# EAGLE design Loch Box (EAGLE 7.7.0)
DESIGNER: A. Stummer; GROUP: A. Steinberg Labs; RELEASE_DATE: 2017 July; REV: A; TITLE: Loch Box; TITLE2: Analog Laser PID

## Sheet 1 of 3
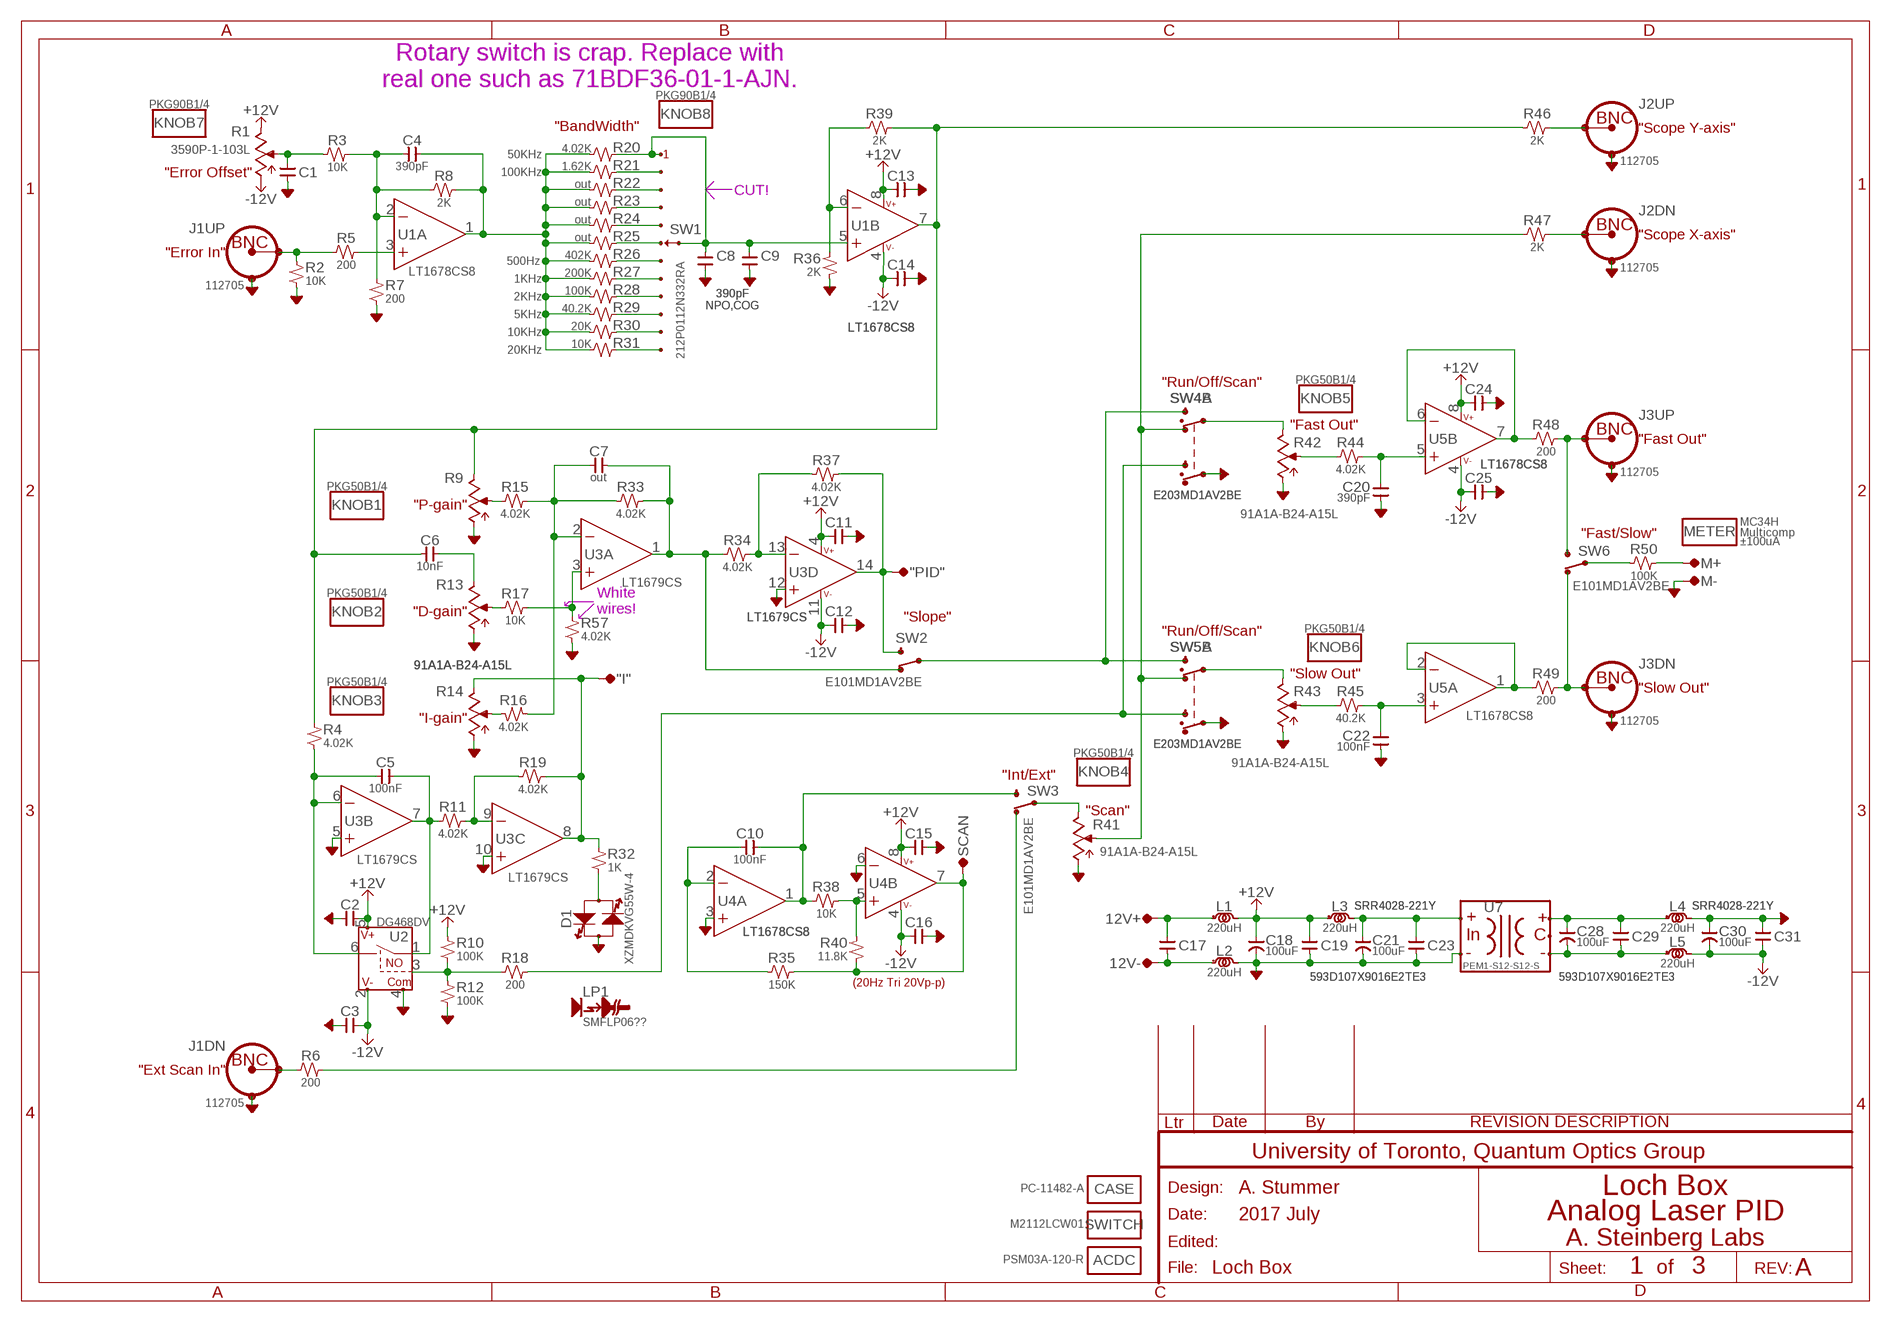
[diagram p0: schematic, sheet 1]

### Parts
12V+  TP-LOOP  [TP-LOOP]
12V-  TP-LOOP  [TP-LOOP]
"I"  TP-0.042B  [TP-0.042B]
"PID"  TP-0.042B  [TP-0.042B]
ACDC  PSM03A-120-R  MISC  [MISC]
C1  100nF  CAP-V-0805  [2012(0805)]
C2  100nF  CAP-H-0805  [2012(0805)]
C3  100nF  CAP-H-0805  [2012(0805)]
C4  390pF  CAP-H-0805  [2012(0805)]
C5  100nF  CAP-H-0805  [2012(0805)]
C6  10nF  CAP-H-0805  [2012(0805)]
C7  out  CAP-H-0805  [2012(0805)]
C8  390pF  CAP-V-0805  [2012(0805)]
C9  390pF  CAP-V-0805  [2012(0805)]
C10  100nF  CAP-H-0805  [2012(0805)]
C11  100nF  CAP-H-0805  [2012(0805)]
C12  100nF  CAP-H-0805  [2012(0805)]
C13  100nF  CAP-H-0805  [2012(0805)]
C14  100nF  CAP-H-0805  [2012(0805)]
C15  100nF  CAP-H-0805  [2012(0805)]
C16  100nF  CAP-H-0805  [2012(0805)]
C17  100nF  CAP-V-0805  [2012(0805)]
C18  100uF  CAP-POL-2917(7343)  [2917(7343)]
C19  100nF  CAP-V-0805  [2012(0805)]
C20  390pF  CAP-V-0805  [2012(0805)]
C21  100uF  CAP-POL-2917(7343)  [2917(7343)]
C22  100nF  CAP-V-0805  [2012(0805)]
C23  100nF  CAP-V-0805  [2012(0805)]
C24  100nF  CAP-H-0805  [2012(0805)]
C25  100nF  CAP-H-0805  [2012(0805)]
C28  100uF  CAP-POL-2917(7343)  [2917(7343)]
C29  100nF  CAP-V-0805  [2012(0805)]
C30  100uF  CAP-POL-2917(7343)  [2917(7343)]
C31  100nF  CAP-V-0805  [2012(0805)]
CASE  PC-11482-A  MISC  [MISC]
D1  XZMDKVG55W-4  LED,DUAL(BIPOLAR)-1206  [1206(3216)]
J1  112705  CONN:BNC,DUAL-112705_ETC  [CONN:BNC,DUAL(BOMAR)]
J2  112705  CONN:BNC,DUAL-112705_ETC  [CONN:BNC,DUAL(BOMAR)]
J3  112705  CONN:BNC,DUAL-112705_ETC  [CONN:BNC,DUAL(BOMAR)]
KNOB1  PKG50B1/4  MISC  [MISC]
KNOB2  PKG50B1/4  MISC  [MISC]
KNOB3  PKG50B1/4  MISC  [MISC]
KNOB4  PKG50B1/4  MISC  [MISC]
KNOB5  PKG50B1/4  MISC  [MISC]
KNOB6  PKG50B1/4  MISC  [MISC]
KNOB7  PKG90B1/4  MISC  [MISC]
KNOB8  PKG90B1/4  MISC  [MISC]
L1  220uH  INDUCTOR-WURTH_744  [INDUCTOR:WURTH_74405]
L2  220uH  INDUCTOR-WURTH_744  [INDUCTOR:WURTH_74405]
L3  220uH  INDUCTOR-WURTH_744  [INDUCTOR:WURTH_74405]
L4  220uH  INDUCTOR-WURTH_744  [INDUCTOR:WURTH_74405]
L5  220uH  INDUCTOR-WURTH_744  [INDUCTOR:WURTH_74405]
LP1  SMFLP06??  LIGHTPIPE-BIVAR_SMFLP  [LIGHTPIPE,BIVAR_SMFLP]
M+  TP-0.042B  [TP-0.042B]
M-  TP-0.042B  [TP-0.042B]
METER  MC34H  MISC  [MISC]
R1  3590P-1-103L  POT-3590  [BOURNS_3590]
R2  10K  R-V-0805  [2012(0805)]
R3  10K  R-H-0805  [2012(0805)]
R4  4.02K  R-V-0805  [2012(0805)]
R5  200  R-H-0805  [2012(0805)]
R6  200  R-H-0805  [2012(0805)]
R7  200  R-V-0805  [2012(0805)]
R8  2K  R-H-0805  [2012(0805)]
R9  91A1A-B24-A15L  POT-BOURNS_91  [BOURNS_91]
R10  100K  R-V-0805  [2012(0805)]
R11  4.02K  R-H-0805  [2012(0805)]
R12  100K  R-V-0805  [2012(0805)]
R13  91A1A-B24-A15L  POT-BOURNS_91  [BOURNS_91]
R14  91A1A-B24-A15L  POT-BOURNS_91  [BOURNS_91]
R15  4.02K  R-H-0805  [2012(0805)]
R16  4.02K  R-H-0805  [2012(0805)]
R17  10K  R-H-0805  [2012(0805)]
R18  200  R-H-0805  [2012(0805)]
R19  4.02K  R-H-0805  [2012(0805)]
R20  4.02K  R-H-0805  [2012(0805)]
R21  1.62K  R-H-0805  [2012(0805)]
R22  out  R-H-0805  [2012(0805)]
R23  out  R-H-0805  [2012(0805)]
R24  out  R-H-0805  [2012(0805)]
R25  out  R-H-0805  [2012(0805)]
R26  402K  R-H-0805  [2012(0805)]
R27  200K  R-H-0805  [2012(0805)]
R28  100K  R-H-0805  [2012(0805)]
R29  40.2K  R-H-0805  [2012(0805)]
R30  20K  R-H-0805  [2012(0805)]
R31  10K  R-H-0805  [2012(0805)]
R32  1K  R-V-0805  [2012(0805)]
R33  4.02K  R-H-0805  [2012(0805)]
R34  4.02K  R-H-0805  [2012(0805)]
R35  150K  R-H-0805  [2012(0805)]
R36  2K  R-V-0805  [2012(0805)]
R37  4.02K  R-H-0805  [2012(0805)]
R38  10K  R-H-0805  [2012(0805)]
R39  2K  R-H-0805  [2012(0805)]
R40  11.8K  R-V-0805  [2012(0805)]
R41  91A1A-B24-A15L  POT-BOURNS_91  [BOURNS_91]
R42  91A1A-B24-A15L  POT-BOURNS_91  [BOURNS_91]
R43  91A1A-B24-A15L  POT-BOURNS_91  [BOURNS_91]
R44  4.02K  R-H-0805  [2012(0805)]
R45  40.2K  R-H-0805  [2012(0805)]
R46  2K  R-H-0805  [2012(0805)]
R47  2K  R-H-0805  [2012(0805)]
R48  200  R-H-0805  [2012(0805)]
R49  200  R-H-0805  [2012(0805)]
R50  100K  R-H-0805  [2012(0805)]
R57  4.02K  R-V-0805  [2012(0805)]
SCAN  TP-0.042B  [TP-0.042B]
SW1  212P0112N332RA  SWITCH,SP12T-CTS_212P0112  [SWITCH,CTS_SP12T(212P0112)]
SW2  E101MD1AV2BE  SWITCH:SPDT-ESWITCH_1??AV2?  [SWITCH:E-SWITCH_1??AV2?]
SW3  E101MD1AV2BE  SWITCH:SPDT-ESWITCH_1??AV2?  [SWITCH:E-SWITCH_1??AV2?]
SW4  E203MD1AV2BE  SWITCH:DPDT-ESWITCH_2??D?AV2?  [SWITCH:E-SWITCH_2??D?AV2?]
SW5  E203MD1AV2BE  SWITCH:DPDT-ESWITCH_2??D?AV2?  [SWITCH:E-SWITCH_2??D?AV2?]
SW6  E101MD1AV2BE  SWITCH:SPDT-ESWITCH_1??AV2?  [SWITCH:E-SWITCH_1??AV2?]
SWITCH  M2112LCW01  MISC  [MISC]
U1  LT1678CS8  OPAMP:AD8___(DUAL)-SOIC-8  [SOIC-8]
U2  DG468DV  SWITCH,ANALOG,SPST,BIPOLAR-TSOP6  [TSOP-6]
U3  LT1679CS  OPAMP,QUAD-SO14  [SOIC-14]
U4  LT1678CS8  OPAMP:AD8___(DUAL)-SOIC-8  [SOIC-8]
U5  LT1678CS8  OPAMP:AD8___(DUAL)-SOIC-8  [SOIC-8]
U7  PEM1-S12-S12-S  DC-DC:DCH01(ISO,UNI/BI,1W)  [DC-DC:DCH01(ISO,UNI/BI,1W)]

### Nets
+12V [power]: C2.1 C11.1 C13.1 C15.1 C18.+(POS) C19.2 C24.1 L1.2(B) L3.1(A) R1.CW R10.2 U1.8(PWR:V++) U2.5(V+) U3.4(V++) U4.8(PWR:V++) U5.8(PWR:V++)
-12V [power]: C3.1 C12.1 C14.1 C16.1 C25.1 C30.-(NEG) C31.1 L5.2(B) R1.CCW U1.4(PWR:V-) U2.2(V-) U3.11(V-) U4.4(PWR:V-) U5.4(PWR:V-)
AGND: C1.1 C2.2 C3.2 C8.1 C9.1 C11.2 C12.2 C13.2 C14.2 C15.2 C16.2 C18.-(NEG) C19.1 C20.1 C21.-(NEG) C22.1 C23.1 C24.2 C25.2 C30.+(POS) C31.2 D1.ONE J1.LWR-COM(DN:SHIELD2) J1.UPR-COM(UP:SHIELD2) J2.LWR-COM(DN:SHIELD2) J2.UPR-COM(UP:SHIELD2) J3.LWR-COM(DN:SHIELD2) J3.UPR-COM(UP:SHIELD2) L2.2(B) L4.2(B) M-.TP R2.1 R7.1 R9.CCW R12.1 R13.CCW R14.CCW R36.1 R41.CCW R42.CCW R43.CCW R57.1 SW4.COM2(B:COM) SW5.COM2(B:COM) U2.4(COM) U3.5(B:+IN) U3.10(C:+IN) U3.12(D:+IN) U4.3(A:+IN) U4.6(B:-IN) U7.IN-
N$1: J1.UPR-CTR(UP:CONDUCTOR) R2.2 R5.1
N$2: R5.2 U1.3(A:+IN)
N$3: C4.1 R3.2 R7.2 R8.1 U1.2(A:-IN)
N$4: C1.2 R1.W R3.1
N$5: C4.2 R8.2 R20.1 R21.1 R22.1 R23.1 R24.1 R25.1 R26.1 R27.1 R28.1 R29.1 R30.1 R31.1 U1.1(A:OUT)
N$6: C6.1 R4.2 R9.CW R39.2 R46.1 U1.7(B:OUT)
N$7: R31.2 SW1.12
N$8: R30.2 SW1.11
N$9: R29.2 SW1.10
N$10: R28.2 SW1.9
N$11: R27.2 SW1.8
N$12: R26.2 SW1.7
N$13: R25.2 SW1.6
N$14: R24.2 SW1.5
N$15: R23.2 SW1.4
N$16: R22.2 SW1.3
N$17: R21.2 SW1.2
N$18: C8.2 C9.2 R20.2 SW1.1 SW1.D(W) U1.5(B:+IN)
N$19: J2.UPR-CTR(UP:CONDUCTOR) R46.2
N$20: R36.2 R39.1 U1.6(B:-IN)
N$21: R9.WIPER(W) R15.1
N$22: R13.WIPER(W) R17.1
N$23: C6.2 R13.CW
N$24: SW2.COM SW4.UP1(A:NO\UP\RIGHT) SW5.UP1(A:NO\UP\RIGHT)
N$25: C7.2 R33.2 R34.1 SW2.DOWN(NC\DOWN\LEFT) U3.1(A:OUT)
N$26: R34.2 R37.1 U3.13(D:-IN)
N$27: C7.1 R15.2 R16.1 R33.1 U3.2(A:-IN)
N$28: "PID".TP R37.2 SW2.UP(NO\UP\RIGHT) U3.14(D:OUT)
N$29: C5.1 R4.1 U2.6(SW2) U3.6(B:-IN)
N$30: C5.2 R11.1 U2.1(SW1) U3.7(B:OUT)
N$31: R11.2 R19.1 U3.9(C:-IN)
N$32: "I".TP R14.CW R19.2 R32.2 U3.8(C:OUT)
N$33: R18.2 SW4.UP2(B:NO\UP\RIGHT) SW5.UP2(B:NO\UP\RIGHT)
N$34: R14.WIPER(W) R16.2
N$35: R41.WIPER(W) R47.1 SW4.DN1(A:NC\DOWN\LEFT) SW5.DN1(A:NC\DOWN\LEFT)
N$36: R42.CW SW4.COM1(A:COM)
N$37: R48.1 U5.6(B:-IN) U5.7(B:OUT)
N$38: R42.WIPER(W) R44.1
N$39: C20.2 R44.2 U5.5(B:+IN)
N$40: J3.UPR-CTR(UP:CONDUCTOR) R48.2 SW6.UP(NO\UP\RIGHT)
N$41: R10.1 R12.2 R18.1 U2.3(IN)
N$42: R38.2 R40.2 U4.5(B:+IN)
N$43: R43.CW SW5.COM1(A:COM)
N$44: R49.1 U5.1(A:OUT) U5.2(A:-IN)
N$45: R43.WIPER(W) R45.1
N$46: C22.2 R45.2 U5.3(A:+IN)
N$47: J3.LWR-CTR(DN:CONDUCTOR) R49.2 SW6.DOWN(NC\DOWN\LEFT)
N$48: C10.1 R35.1 U4.2(A:-IN)
N$49: R41.CW SW3.COM
N$50: J1.LWR-CTR(DN:CONDUCTOR) R6.1
N$51: C10.2 R38.1 SW3.UP(NO\UP\RIGHT) U4.1(A:OUT)
N$52: R50.1 SW6.COM
N$53: R6.2 SW3.DOWN(NC\DOWN\LEFT)
N$54: J2.LWR-CTR(DN:CONDUCTOR) R47.2
N$55: R35.2 R40.1 SCAN.TP U4.7(B:OUT)
N$56: M+.TP R50.2
N$57: D1.T'OTHER R32.1
N$58 [power]: 12V-.P$1(TP) C17.1 L2.1(A)
N$59 [power]: C28.+(POS) C29.2 L4.1(A) U7.OUT+
N$60 [power]: C21.+(POS) C23.2 L3.2(B) U7.IN+
N$62 [power]: 12V+.P$1(TP) C17.2 L1.1(A)
N$64 [power]: C28.-(NEG) C29.1 L5.1(A) U7.OUT-
N$69: R17.2 R57.2 U3.3(A:+IN)
Unconnected: SW4.DN2(B:NC\DOWN\LEFT) SW5.DN2(B:NC\DOWN\LEFT) U7.COM

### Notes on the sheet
- Rotary switch is crap. Replace with
  real one such as 71BDF36-01-1-AJN.
- "Scope Y-axis"
- 50KHz
- "Error Offset" | 100KHz
- CUT!
- "Scope X-axis"
- "Error In"
- 500Hz
- 1KHz
- 2KHz
- 5KHz
- 10KHz
- 20KHz
- "Fast Out"
- White
  wires!
- "Slow Out"
- NO
- (20Hz Tri 20Vp-p)
- "Ext Scan In"

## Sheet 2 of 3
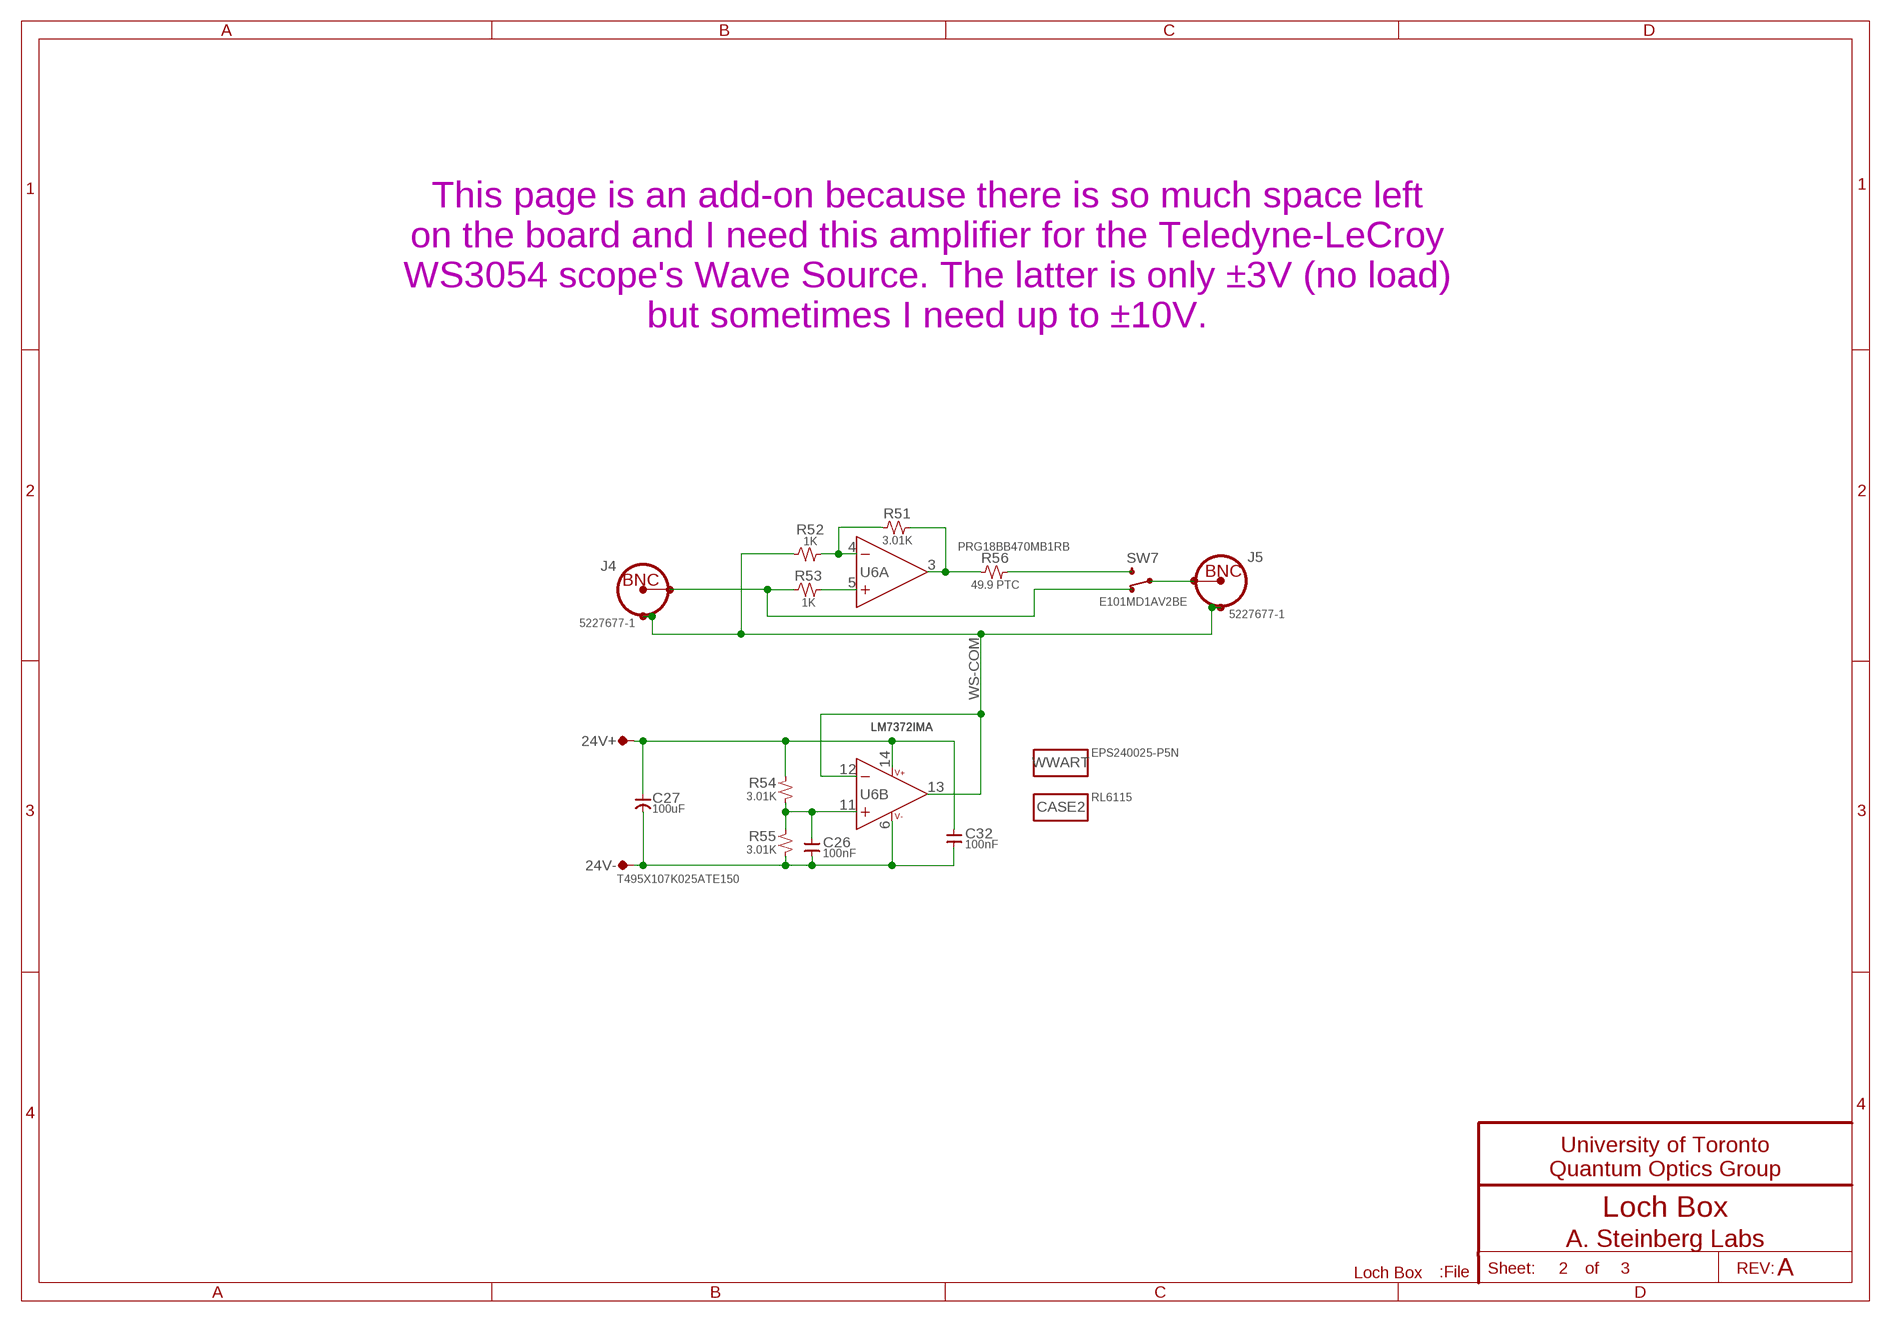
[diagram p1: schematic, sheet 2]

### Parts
24V+  TP-LOOP  [TP-LOOP]
24V-  TP-LOOP  [TP-LOOP]
C26  100nF  CAP-V-0805  [2012(0805)]
C27  100uF  CAP-POL-2917(7343)  [2917(7343)]
C32  100nF  CAP-V-0805  [2012(0805)]
CASE2  RL6115  MISC  [MISC]
J4  5227677-1  CONN:BNCTYPE3HORIZ  [CONN:BNC-AMP-TYPE3HORIZ]
J5  5227677-1  CONN:BNCTYPE3HORIZ  [CONN:BNC-AMP-TYPE3HORIZ]
R51  3.01K  R-H-0805  [2012(0805)]
R52  1K  R-H-0805  [2012(0805)]
R53  1K  R-H-0805  [2012(0805)]
R54  3.01K  R-V-0805  [2012(0805)]
R55  3.01K  R-V-0805  [2012(0805)]
R56  49.9 PTC  R-H-0805  [2012(0805)]
SW7  E101MD1AV2BE  SWITCH:SPDT-ESWITCH_1??AV2?  [SWITCH:E-SWITCH_1??AV2?]
U6  LM7372IMA  OPAMP_DUAL-SOIC16#1  [SOIC-16]
WWART  EPS240025-P5N  MISC  [MISC]

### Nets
N$63: R51.1 R52.2 U6.4(A:-IN)
N$65: R56.2 SW7.UP(NO\UP\RIGHT)
N$66: J5.CONDUCTOR SW7.COM
N$67: J4.CONDUCTOR R53.1 SW7.DOWN(NC\DOWN\LEFT)
N$68: R53.2 U6.5(A:+IN)
N$70: C26.2 R54.1 R55.2 U6.11(B:+IN)
N$71: 24V-.P$1(TP) C26.1 C27.-(NEG) C32.1 R55.1 U6.6(.:V-)
N$72: 24V+.P$1(TP) C27.+(POS) C32.2 R54.2 U6.14(.:V++)
N$74: R51.2 R56.1 U6.3(A:OUT)
WS-COM: J4.SHIELD1 J4.SHIELD2 J5.SHIELD1 J5.SHIELD2 R52.1 U6.12(B:-IN) U6.13(B:OUT)

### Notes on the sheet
- This page is an add-on because there is so much space left
  on the board and I need this amplifier for the Teledyne-LeCroy
  WS3054 scope's Wave Source. The latter is only ±3V (no load)
  but sometimes I need up to ±10V.

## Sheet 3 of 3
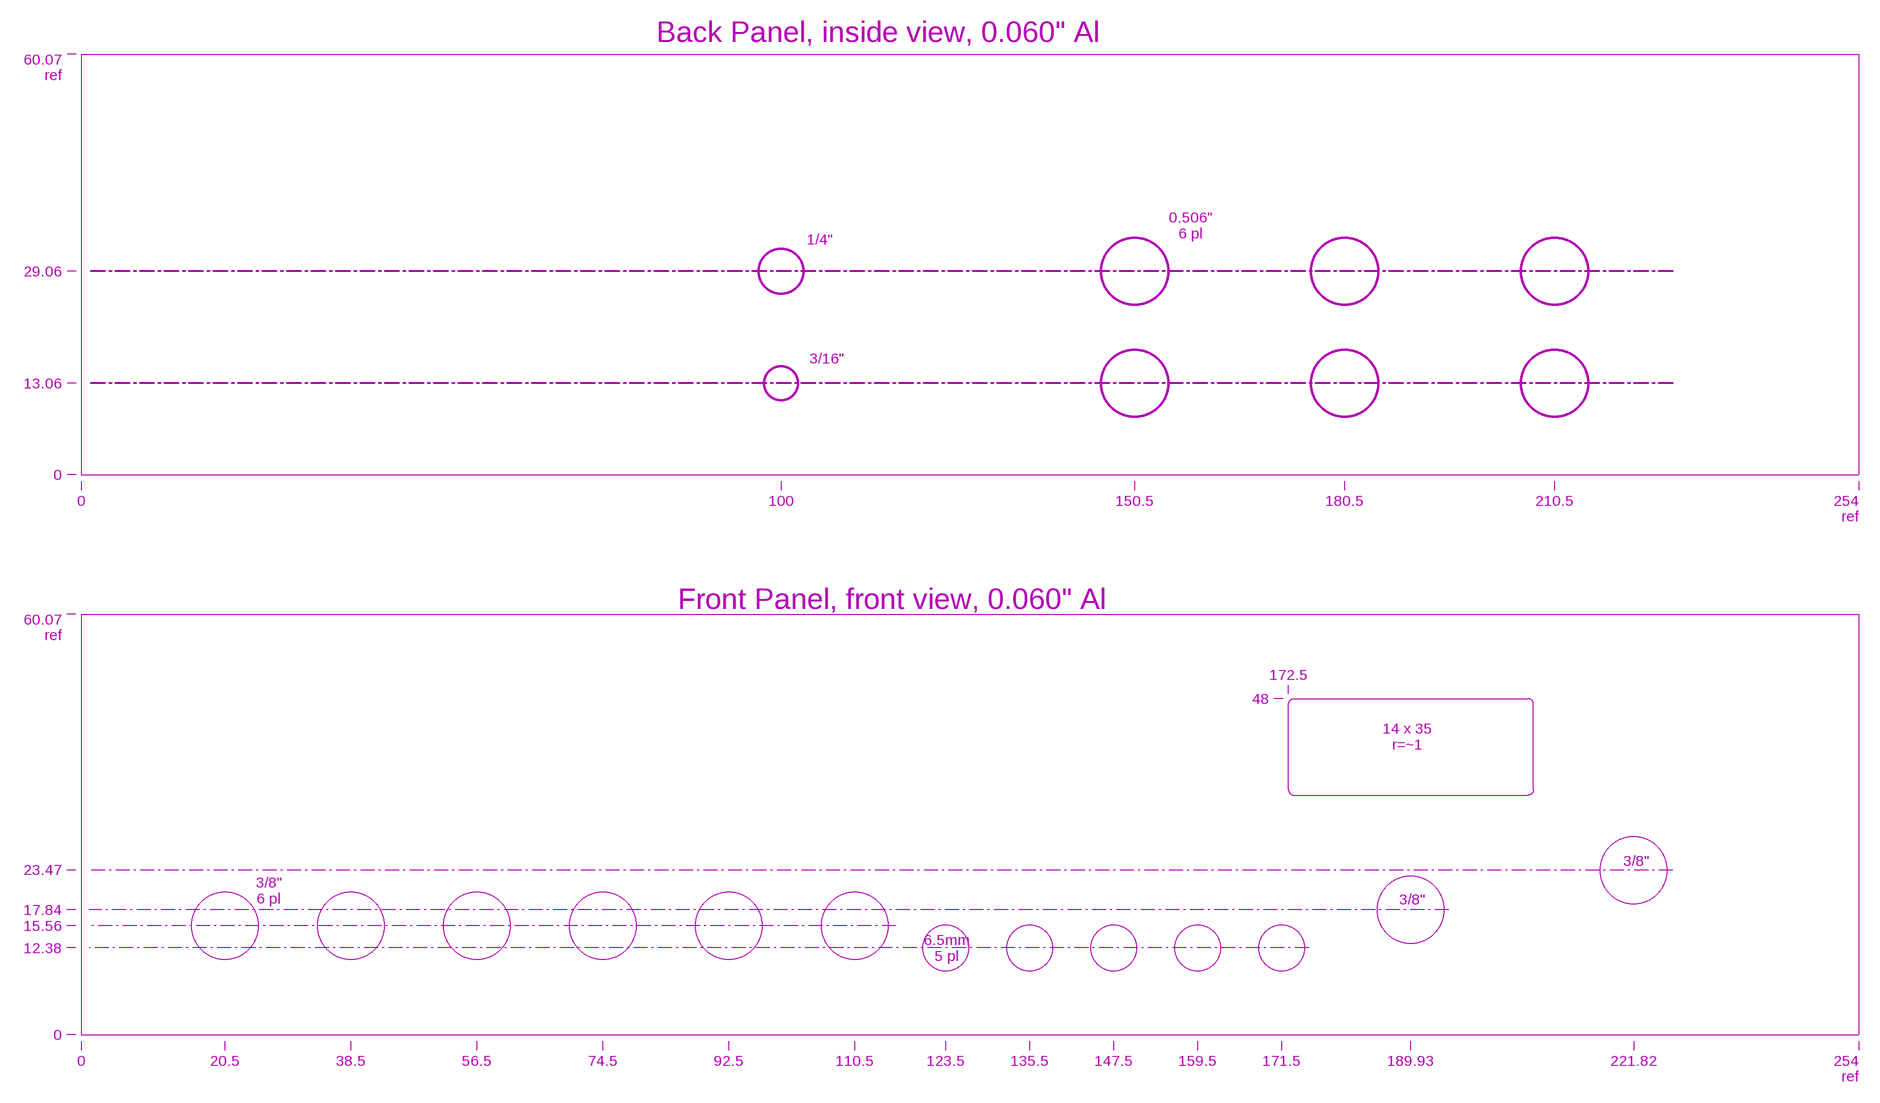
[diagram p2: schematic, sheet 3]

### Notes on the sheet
- Back Panel, inside view, 0.060" Al
- 60.07
  ref
- 0.506"
  6 pl
- 1/4"
- 29.06
- 3/16"
- 13.06
- 0
- 0 | 100 | 150.5 | 180.5 | 210.5
- 254
  ref
- Front Panel, front view, 0.060" Al
- 60.07
  ref
- 172.5
- 48
- 14 x 35
  r=~1
- 3/8"
- 23.47
- 3/8"
  6 pl
- 3/8"
- 17.84
- 15.56
- 6.5mm
  5 pl
- 12.38
- 0
- 0 | 20.5 | 38.5 | 56.5 | 74.5 | 92.5 | 110.5 | 123.5 | 135.5 | 147.5 | 159.5 | 171.5 | 189.93 | 221.82
- 254
  ref

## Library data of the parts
12V+ 12V- 24V+ 24V- "I" "PID" M+ M- SCAN = QuantumOptics:TP: Testpoint, single pin or single socket, either SMT pad, small hole or loop style TP such as Keystone 5002K (0.042").
ACDC CASE CASE2 KNOB1-KNOB8 SWITCH WWART = QuantumOptics:MISC: Miscellaneous Part, just a placeholder for miscellaeous parts
C1 C17 C19 C20 C22 C23 C26 C29 C31 C32 = QuantumOptics:CAP-V-: Cap, SMT and Through-hole, 0402 and up.
C2-C7 C10-C16 C24 C25 = QuantumOptics:CAP-H-: Cap, SMT and Through-hole, 0402 and up.
C8 C9 = QuantumOptics:CAP-V-: Cap, SMT and Through-hole, 0402 and up.; TEMPCO: NPO,COG
C18 C21 C28 C30 = QuantumOptics:CAP-POL-: Capacitor, Polarized, SMT 0805 and up, probably tantalum.; PN: 593D107X9016E2TE3
C27 = QuantumOptics:CAP-POL-: Capacitor, Polarized, SMT 0805 and up, probably tantalum.; PN: T495X107K025ATE150
D1 = QuantumOptics:LED,DUAL(BIPOLAR): LED, dual biploar such as SunLED XZMDKVG55W-4.
J1-J3 = QuantumOptics:CONN:BNC,DUAL: Dual BNC, panel mount RA throughhole, Isolated: Amphenol 31-657 and 112705/6. Sheilds connected: Amphenol 031-6578, Cinch VBI501 (cheapest) and Bomar 364A2595.; NUT: 1-1634816-0
J4 J5 = QuantumOptics:CONN:BNC: BNC PCB, horizontal or vertical, e.g. Horiz: Amp (5)227677-1, nut 1-329631-2, shoulder washer 330620, vert isolated 5227222-6, http://catalog.tycoelectronics.com/TE/bin/TE.Connect?C=1&M=BYPN&TCPN=5227222-6&RQPN=5227222-6 ...
L1-L5 = QuantumOptics:INDUCTOR: Inductor, generic inductor.; PN: SRR4028-221Y
LP1 = QuantumOptics:LIGHTPIPE: Lightpipe for SMT LEDs
METER = QuantumOptics:MISC: Miscellaneous Part, just a placeholder for miscellaeous parts; MFG: Multicomp; RANGE: ±100uA
R1 = QuantumOptics:POT: Pot, regular or trimpot
R2 R4 R7 R10 R12 R32 R36 R40 R54 R55 R57 = QuantumOptics:R-V-*: Resistor, SMT & Through-Hole, vertical symbol
R3 R5 R6 R8 R11 R15-R31 R33-R35 R37-R39 R44-R53 = QuantumOptics:R-H-*: Resistor, SMT & Through-Hole, horizontal symbol
R9 = QuantumOptics:POT: Pot, regular or trimpot; DESC: "P-gain"
R13 = QuantumOptics:POT: Pot, regular or trimpot; DESC: "D-gain"
R14 = QuantumOptics:POT: Pot, regular or trimpot; DESC: "I-gain"
R41 = QuantumOptics:POT: Pot, regular or trimpot; DESC: "Scan"
R42 = QuantumOptics:POT: Pot, regular or trimpot; DESC: "Fast Out"
R43 = QuantumOptics:POT: Pot, regular or trimpot; DESC: "Slow Out"
R56 = QuantumOptics:R-H-*: Resistor, SMT & Through-Hole, horizontal symbol; PN: PRG18BB470MB1RB
SW1 = QuantumOptics:SWITCH,SP12T: Switch, SP12T, can be part of DP12T, can have stops to reduce positions.; DESC: "BandWidth"
SW2 = QuantumOptics:SWITCH:SPDT: Switch, SPDT; DESC: "Slope"
SW3 = QuantumOptics:SWITCH:SPDT: Switch, SPDT; DESC: "Int/Ext"
SW4 SW5 = QuantumOptics:SWITCH:DPDT: Switch, DPDT; DESC: "Run/Off/Scan"
SW6 = QuantumOptics:SWITCH:SPDT: Switch, SPDT; DESC: "Fast/Slow"
SW7 = QuantumOptics:SWITCH:SPDT: Switch, SPDT
U1 U4 U5 = QuantumOptics:OPAMP:AD8___(DUAL): AD8xxx, Analog Devices, dual opamp in SOIC-8 and MSOP-8, various versions available. AD8066, AD8656, etc. e.g. http://www.analog.com/UploadedFiles/Data_Sheets/476080131AD8655_6_a.pdf
U2 = QuantumOptics:SWITCH,ANALOG,SPST,BIPOLAR: Analog SPST switch, bipolar such as Vishay DG467/8
U3 = QuantumOptics:OPAMP,QUAD: Quad opamp, such as LT1679 or LT1491
U6 = QuantumOptics:OPAMP_DUAL: Dual Op Amp, common pinouts. Based on http://www.analog.com/static/imported-files/data_sheets/AD8651_8652.pdf
U7 = QuantumOptics:DC-DC:DCH01(ISO,UNI/BI,1W): DC-DC DCH01, TI, isolated, unregulated, uni- bipolar. http://focus.ti.com/lit/ds/symlink/dch010505d.pdf; MFG: TI

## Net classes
0 default: width 0.152 mm, drill 0.254 mm, clearance 0.152 mm
1 power: width 0.635 mm, drill 0.254 mm, clearance 0.254 mm

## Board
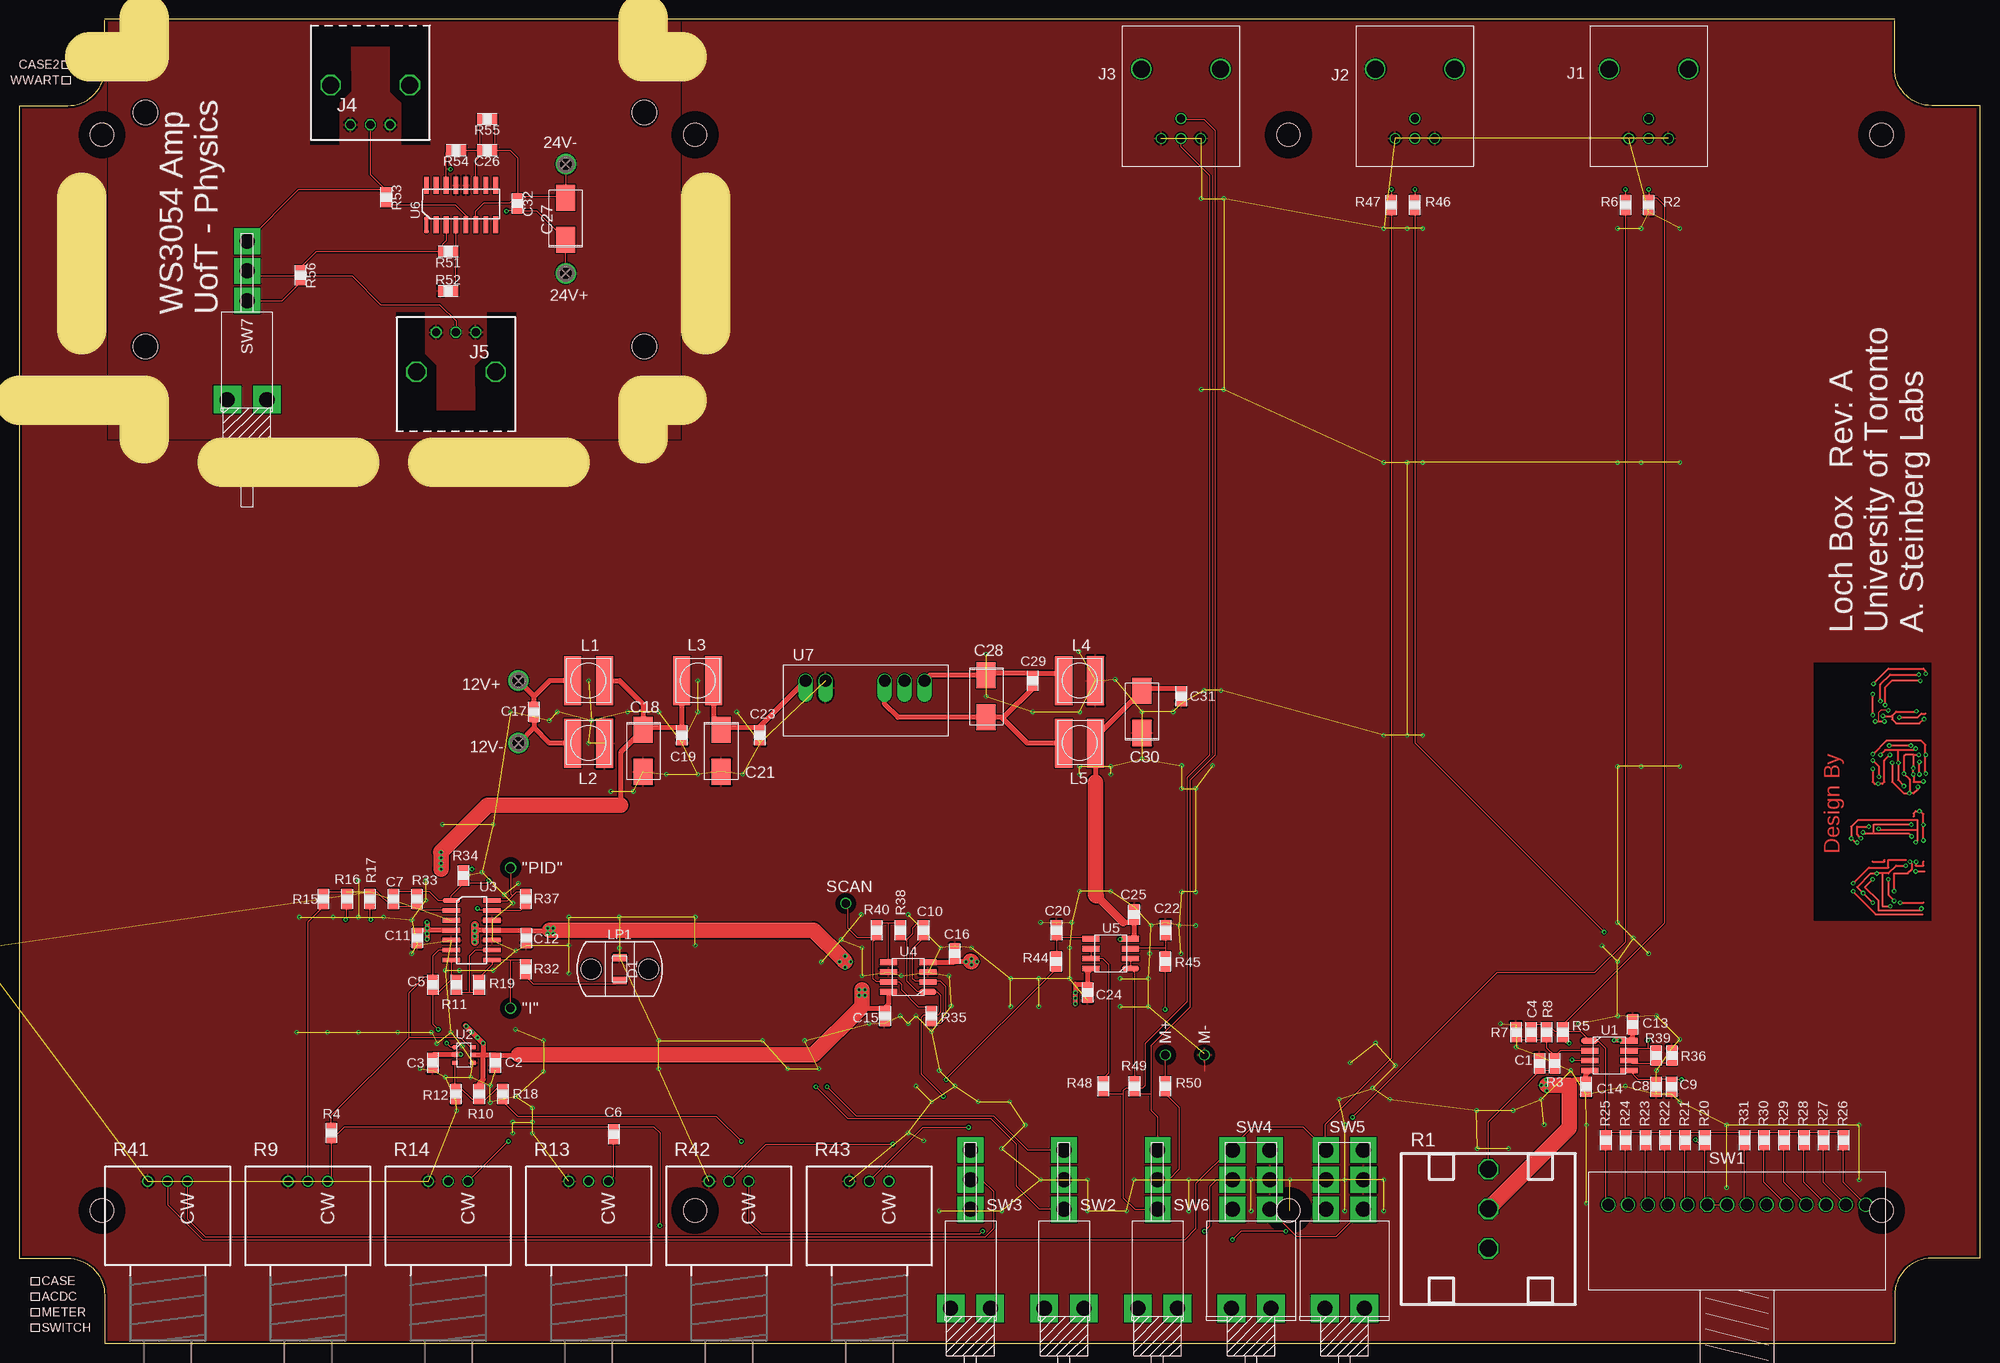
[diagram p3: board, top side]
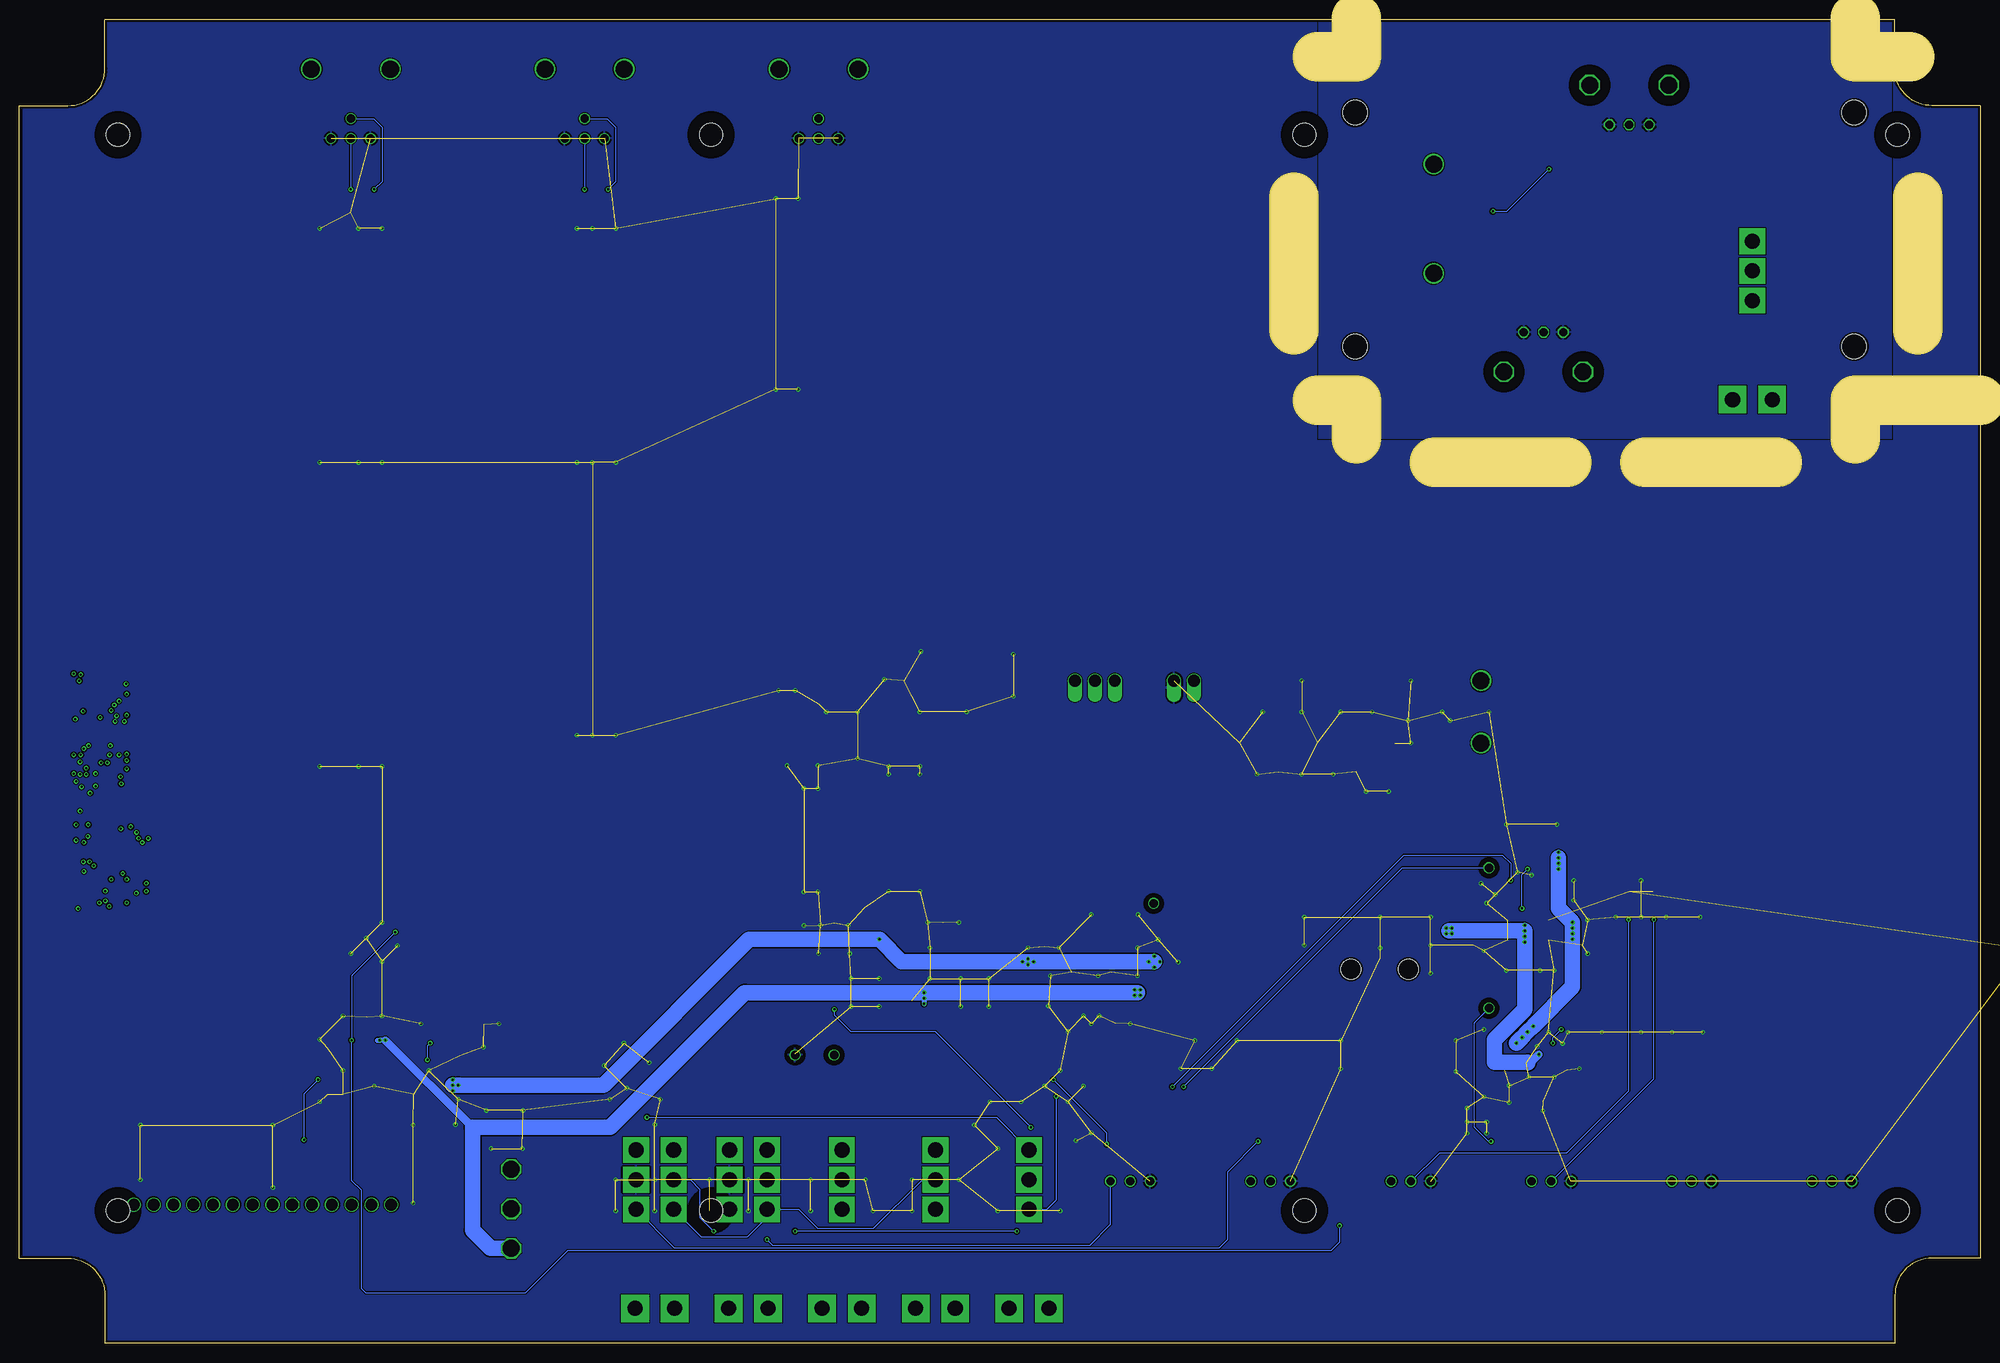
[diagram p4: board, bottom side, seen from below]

Size 251.5 x 169.8 mm. Coordinates in mm from the lower left corner, seen from the top.
Copper layers (1+16): Top 0.04318125mm / dielectric 7.5mil / Bottom 0.04318125mm
Design rules "~DRC for PCBWay, 2-layer #1, 6&6mil & 0.3mm drill": minimum track width 6mil, minimum drill 0.25mm, track to track 6mil, track to pad 6mil, pad to pad 6mil, via to via 6mil, smd to smd 0mil, copper to edge 10mil, drill to drill 6mil, minimum pad ring 6mil, minimum via ring 6mil, stop-mask expansion 4mil, vias tented up to drill 0mil, thermal gap 10mil
Holes 3.17 mm at 16.14,127.85 16.14,157.85 80.15,157.85 80.15,127.85
tRestrict: 4 lines
Milling: 12 lines

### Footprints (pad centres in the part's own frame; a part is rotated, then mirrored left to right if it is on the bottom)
TP-LOOP = drill 2.184 pad 2.54: P$1 0,0
TP-0.042B = drill 1.092: TP 0,0
2012(0805) = smd 0.7 x 1.3: 1 -0.95,0; 2 0.95,0
2917(7343) = smd 3.35 x 2.45: + -2.7,0; - 2.7,0
1206(3216) = smd 0.9 x 1.7: ONE -1.45,0; T'OTHER 1.45,0
CONN:BNC,DUAL(BOMAR) = drill 1.067: LWR-COM 14.45,-2.54; LWR-CTR 11.91,0; UPR-COM 14.45,2.54; UPR-CTR 14.45,0 | drill 2.184: MTG1 5.56,-5.08; MTG2 5.56,5.08
CONN:BNC-AMP-TYPE3HORIZ = drill 1.067 octagon: CONDUCTOR 0,-12.7; SHIELD1 -2.54,-12.7; SHIELD2 2.54,-12.7 | drill 2.184 octagon: P$1 -5.08,-7.62; P$2 5.08,-7.62
INDUCTOR:WURTH_74405 = smd 6.3 x 2.2: 1 0,2.05; 2 0,-2.05
LIGHTPIPE,BIVAR_SMFLP = hole 2.578: -3.683,0; 3.683,0
BOURNS_3590 = drill 2.184 octagon: CCW -12.065,0; CW -6.985,0; W -17.145,0
BOURNS_91 = drill 1.067: CCW -10.795,-2.54; CW -10.795,2.54; WIPER -10.795,0
SWITCH,CTS_SP12T(212P0112) = drill 1.5: 1 0,-1.27; 2 0,-6.35; 3 0,-8.89; 4 0,-11.43; 5 0,-13.97; 6 0,-16.51; 7 0,16.51; 8 0,13.97; 9 0,11.43; 10 0,8.89; 11 0,6.35; 11.5 0,3.81; 12 0,1.27 | drill 1.5 octagon: D 0,-3.81
SWITCH:E-SWITCH_1??AV2? = drill 1.93 pad 3.302 square: COM 0,0; DOWN -3.81,0; UP 3.81,0 | drill 1.93 pad 3.556 square: MTG1 16.51,-2.54; MTG2 16.51,2.54
SWITCH:E-SWITCH_2??D?AV2? = drill 1.93 pad 3.302 square: COM1 0,-2.413; COM2 0,2.413; DN1 -3.81,-2.413; DN2 -3.81,2.413; UP1 3.81,-2.413; UP2 3.81,2.413 | drill 1.93 pad 3.556 square: MTG1 16.51,-2.54; MTG2 16.51,2.54
SOIC-8 = smd 0.75 x 2.2: 1 -1.905,-2.532; 2 -0.635,-2.532; 3 0.635,-2.532; 4 1.905,-2.532; 5 1.905,2.532; 6 0.635,2.532; 7 -0.635,2.532; 8 -1.905,2.532
TSOP-6 = smd 0.508 x 0.711: 1 -0.991,-1.168; 2 0,-1.168; 3 0.991,-1.168; 4 0.991,1.168; 5 0,1.168; 6 -0.991,1.168
SOIC-14 = smd 0.6 x 2.2: 1 -3.81,-2.6; 2 -2.54,-2.6; 3 -1.27,-2.6; 4 0,-2.6; 5 1.27,-2.6; 6 2.54,-2.6; 7 3.81,-2.6; 8 3.81,2.6; 9 2.54,2.6; 10 1.27,2.6; 11 0,2.6; 12 -1.27,2.6; 13 -2.54,2.6; 14 -3.81,2.6
SOIC-16 = smd 0.6 x 2.2: 1 -3.81,-2.54; 2 -2.54,-2.54; 3 -1.27,-2.54; 4 0,-2.54; 5 1.27,-2.54; 6 2.54,-2.54; 7 3.81,-2.54; 8 5.08,-2.54; 9 5.08,2.54; 10 3.81,2.54; 11 2.54,2.54; 12 1.27,2.54; 13 0,2.54; 14 -1.27,2.54; 15 -2.54,2.54; 16 -3.81,2.54
DC-DC:DCH01(ISO,UNI/BI,1W) = drill 1.524 offset: COM 2.54,0; IN+ -10.16,0; IN- -7.62,0; OUT+ 5.08,0; OUT- 0,0
CASE,BUD_PC11482 = hole 3: 10.582,17.056; 86.681,17.056; 162.779,17.056; 238.878,17.056; 10.582,155.029; 86.681,155.029; 162.779,155.029; 238.878,155.029

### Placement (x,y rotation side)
12V+  64,85 0 top
12V-  64,77 0 top
24V+  70.08,137.24 180 top
24V-  70.08,151.24 0 top
"I"  63,43 0 top
"PID"  63,61 0 top
ACDC  2,6 0 top
C1  194.96,35.92 270 top
C2  61,36 270 top
C3  53,36 270 top
C4  193.96,39.92 90 top
C5  53,46 270 top
C6  76.21,26.84 270 top
C7  48,57 90 top
C8  209.96,32.92 90 top
C9  211.96,32.92 90 top
C10  116,53 90 top
C11  51,52 270 top
C12  65,52 270 top
C13  206.96,40.92 90 top
C14  200.96,32.92 270 top
C15  111,42 270 top
C16  120,50 90 top
C17  66,81 90 top
C18  80,76 270 top
C19  85,78 90 top
C20  133,53 270 top
C21  90,76 270 top
C22  147,53 270 top
C23  95,78 90 top
C24  137,45 270 top
C25  143,55 90 top
C26  60,153 180 top
C27  70.08,144.24 90 top
C28  124,83 270 top
C29  130,85 90 top
C30  144,81 90 top
C31  149,83 270 top
C32  63.84,146.2 270 top
CASE  2,8 0 top
CASE2  6,164 180 top
D1  77,48 270 top
J1  209,169 270 top
J2  179,169 270 top
J3  149,169 270 top
J4  45,169 0 top
J5  56,117 180 top
KNOB1  not placed on the board
KNOB2  not placed on the board
KNOB3  not placed on the board
KNOB4  not placed on the board
KNOB5  not placed on the board
KNOB6  not placed on the board
KNOB7  not placed on the board
KNOB8  not placed on the board
L1  73,85 90 top
L2  73,77 90 top
L3  87,85 90 top
L4  136,85 90 top
L5  136,77 90 top
LP1  77,48 0 top
M+  147,37 90 top
M-  152,37 90 top
METER  2,4 0 top
R1  188.43,5.2 270 top
R2  209,146 90 top
R3  196.96,35.92 90 top
R4  40,27 270 top
R5  197.96,39.92 270 top
R6  206,146 270 top
R7  191.96,39.92 270 top
R8  195.96,39.92 90 top
R9  37,10 270 top
R10  59,32 90 top
R11  56,46 270 top
R12  56,32 90 top
R13  73,10 270 top
R14  55,10 270 top
R15  39,57 90 top
R16  42,57 270 top
R17  45,57 90 top
R18  62,32 270 top
R19  59,46 90 top
R20  216.17,26.05 270 top
R21  213.63,26.05 270 top
R22  211.09,26.05 270 top
R23  208.55,26.05 270 top
R24  206.01,26.05 270 top
R25  203.47,26.05 270 top
R26  233.95,26.05 270 top
R27  231.41,26.05 270 top
R28  228.87,26.05 270 top
R29  226.33,26.05 270 top
R30  223.79,26.05 270 top
R31  221.25,26.05 270 top
R32  65,48 90 top
R33  51,57 90 top
R34  57,60 90 top
R35  117,42 90 top
R36  211.96,36.92 270 top
R37  65,57 90 top
R38  113,53 90 top
R39  209.96,36.92 90 top
R40  110,53 90 top
R41  19,10 270 top
R42  91,10 270 top
R43  109,10 270 top
R44  133,49 90 top
R45  147,49 90 top
R46  179,146 90 top
R47  176,146 90 top
R48  139,33 270 top
R49  143,33 270 top
R50  147,33 90 top
R51  55,140 180 top
R52  55,135 0 top
R53  47,147 270 top
R54  56,153 180 top
R55  60,157 180 top
R56  36,137 270 top
R57  not placed on the board
SCAN  106,56.44 0 top
SW1  220.32,17.8 270 top
SW2  134,21 270 top
SW3  122,21 270 top
SW4  158,21 270 top
SW5  170,21 270 top
SW6  146,21 270 top
SW7  29.2,137.56 270 top
SWITCH  2,2 0 top
U1  203.96,36.92 270 top
U2  57,37 270 top
U3  58,53 270 top
U4  114,47 90 top
U5  140,50 90 top
U6  56,146 0 top
U7  111,85 0 top
U$34  [CASE,HAMMOND_RL6105_RL6115]  85,116 90 top
U$47  [CASE,BUD_PC11482]  0,0 0 top
WWART  6,162 180 top

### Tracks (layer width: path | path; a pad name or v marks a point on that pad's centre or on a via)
+12V  (via drill 0.25)
  Top 0.635: C13.1 206.96,39.29 U1.8 206.44,38.88 v204.56,38.88 | U5.8 137,47.63 C24.1 136.87,46.08 135.44,46.08 v135.44,45 | U3.4 52.28,53 | 52.28,53 51.05,53 C11.1 | U2.5 59.48,37 | 59.48,37 60.95,37 C2.1 64,36.95 64,37 | L1.2 77,85 80,82 C18.+ | C18.+ 80.25,78.95 C19.2 85,84.95 L3.1 | 111.37,45 U4.8 111.47,43.42 C15.1 107.83,42.95 107.72,42.95 v107.72,45.36 | C18.+ 77.12,75.82 77.12,69.04 | v52.28,54 52.28,53 | 59.48,37 v59.48,38.52 57.2,40.8 | R10.2 59,33.36 59.48,33.84 59.48,37 | v52.28,51.84 v52.28,52.56 52.28,52.92 | v135.44,43.56 v135.44,44.99 | 54.08,60.78 v54.08,60.84 | v107.72,45.36 108.08,45.36 v108.44,45.36 | v108.44,44.64 v107.72,44.64 v107.72,45.36
  Top 2: 107.83,42.95 101.88,37 64,37 | 77.12,69.04 60.04,69.04 54,63 v54.08,63 v54.08,60.84 | 108.08,43.31 108.08,45.36
  Bottom 0.635: v54.08,63 v54.08,62.28 | v135.44,43.56 v135.44,44.28 v135.44,45 | v204.56,38.88 v205.28,38.88 205.57,38.88 | 108.08,45 108.44,45 v108.44,44.64
  Bottom 1: v204.56,38.88 193.4,27.72
  Bottom 2: R1.CW 191.06,12.19 193.4,14.52 193.4,27.72 175.76,27.72 158.48,45 v135.44,45 108.08,45 | v59.48,38.52 v58.76,39.24 v58.04,39.96 v57.32,40.68 52.28,45.72 v52.28,52.56 v52.28,53.28 v52.28,54 54.08,55.8 v54.08,60.84 v54.08,61.56 v54.08,62.28
-12V  (via drill 0.25)
  Top 0.635: U1.4 200.96,34.55 C14.1 199.55,33.87 198.8,33.12 | U4.4 119.86,48.91 C16.1 122.03,49.05 | C3.1 53.05,37 U2.2 55.91,37.08 v56.6,37.08 | C31.1 144.25,83.95 C30.- 138.05,77.75 L5.2 138,77 138,72 | v141.2,51.84 142.47,51.84 U5.4 143,52.37 C25.1 142.95,54 141.56,54 | v122.12,49.32 121.4,49.32 v121.4,48.96 | v122.12,48.6 v122.12,49.32 | v122.84,48.96 122.12,48.96 v122.12,49.32 | v105.92,49.68 105.56,49.68 105.56,49.32 | v105.2,48.96 105.92,48.96 | 105.92,48.96 v105.92,48.24 | 105.92,48.96 v106.64,48.96 | v67.76,53.28 v67.76,52.56 v68.48,52.56 | v67.76,53.28 v68.48,53.28 | v67.76,53.28 68,53.04 68,53 68,52.95 C12.1 64.95,53 U3.11 58.48,53 v58.4,52.92 v58.4,53.64
  Top 1: 138.05,57.51 138.14,57.42 141.56,54 | v58.4,53.64 v58.4,52.2 v58.4,51.48
  Top 2: R1.CCW 198.8,27.64 198.8,33.12 v195.92,33.12 | 122.03,49.05 122.12,48.96 | 105.92,48.96 105.56,49.32 101.88,53 68,53 | 138,72 138,57.56 138.14,57.42
  Bottom 0.635: 122.12,48.96 v122.12,49.32 | v195.92,33.84 v195.92,33.12 v195.92,32.4 | 105.92,48.96 v105.92,49.68 | v58.4,52.92 58.37,52.95 58.37,53.61 v58.4,53.64
  Bottom 1: 58,36 57.68,36 v56.6,37.08
  Bottom 2: v195.92,33.12 v195.2,33.12 176.6,33.12 157.88,51.84 v141.2,51.84 138.32,48.96 122.12,48.96 105.92,48.96 | 58,36 58,36.08 62.28,36.08 62.28,38.96 58.4,42.84 v58.4,52.92 68.12,52.92
AGND  (via drill 0.25)  (261 unrouted)
  Top 0.152: 152,37.16 M-.TP 152,34.92
  other vias: 63,81 69,81 78,81 82,81 87,81 92,81 73,77 73,85 87,85 87,73 83,73 124,83 130,81 136,81 144,81 144,75 148,81 136,73 140,73 136,58 136,74 140,74 140,58 145.16,53.64 148.76,53.64 149,50 145,50 141.2,46.8 144.8,46.8 144.8,43.2 141.2,43.2 134.72,46.8 134.72,50.76 135,54 131,54 130.76,46.8 130.76,43.2 127.16,43.2 127.16,46.8 119.24,47.16 122.12,50.76 118.16,50.76 119.52,43.28 115,42 113,42 114,55 108,55 108.08,50.76 108.08,47.16 113.12,47.16 109,41 114,41 117,40 120,33 115,33 118,35 117,31 114,27 116,26 127,31 126,25 129,28 123,31 118,17 126,17 131,21 137,17 137,21 143,21 142,17 150,17 150,21 158,21 158,17 163,17 163,21 170,21 170,17 175,17 175,21 170,28.08 169.28,31.32 173.6,32.76 175.76,31.32 176.48,35.64 173.96,38.52 170.72,36 186.92,29.88 187,25 191,25 195.56,28.08 201,18 219,20 236,21 236,28 219,28 201,28 206,33 210,35 213,31 213,39 210,42 205,42 200,41 190,41 192,38 199,35 195.2,31.32 191.6,29.88 205,49 207,52 205,54 203,51 209,50 213,74 208,74 205,74 205,113 208,113 213,113 213,143 208,143 205,143 180,143 178,143 175,143 175,113 178,113 180,113 180,78 178,78 175,78 102.52,35.24 98.56,35.24 100.72,38.84 95.32,38.84 67.24,34.88 67.24,38.84 82,38.84 82,35.24 60.4,33.08 57.88,34.16 54.64,34.16 56.08,29.84 60.4,30.92 63.28,28.4 65.8,28.4 65.8,26.96 63.28,26.96 51.4,35.24 53.56,38.48 56.8,38.12 55.36,39.92 52.84,39.92 48.52,39.92 54.64,47.84 56.44,47.84 60.76,47.84 63.64,50.36 70.48,47.48 76.96,50.72 70.48,51.08 70.48,54.68 76.96,54.68 86.68,54.68 86.68,51.08 102.88,48.92 105.4,51.8 63.28,56.48 62.2,57.56 64,59 59.32,60.44 57.52,60.08 52.12,59.36 52.12,56.84 50.32,54.32 50.32,50 46.72,54.68 43.48,54.68 40.24,54.68 43.48,59.36 35.92,54.68 35.56,39.92 39.52,39.92 43.48,39.92 63.64,40.28 63.64,31.64 65.8,30.2 54.28,66.56 60.76,66.56 73.36,79.88 67.96,79.88 75.88,70.8 78.76,70.8 92.76,73 124,88.4 135.88,88.76 140.56,85.16 154.48,146.84 151.6,146.84 151.6,122.36 154.48,122.36 151.96,83.76 154.12,83.76 149.08,71.16 150.88,71.16 149.08,74.12 153.04,74.12 149.08,57.92 150.88,57.92 150.88,53.6
  pour Top (rank 2): 0,0 251,0 251,170 0,170
  pour Bottom (rank 2): 0,0 251,0 251,170 0,170
N$1  (via drill 0.25)
  Top 0.152: v209,148 R2.2 210.05,146.95 211,146 211,53.91 R5.1
  Bottom 0.152: J1.UPR-CTR v209,148
N$2  (via drill 0.25)
  Top 0.152: U1.3 199.24,36.28 v199.16,36.36 | v198.8,38.52 198.41,38.52 R5.2
  Bottom 0.152: v199.16,36.36 199.16,38.16 v198.8,38.52
N$3
  Top 0.152: R7.2 C4.1 R8.1 195.96,37.87 R3.2 197.65,37.55 U1.2
N$4
  Top 0.152: R3.1 C1.2 188.43,28.44 R1.W
N$5
  Top 0.152: C4.2 R8.2 196.09,40.87 197,39.96 200.29,39.96 U1.1 201.48,38.88 202.4,38.88 203.47,37.81 R25.1 R24.1 R23.1 R22.1 R21.1 R20.1 R31.1 R30.1 R29.1 R28.1 R27.1 R26.1
N$6  (via drill 0.25)
  Top 0.152: U1.7 206.81,37.87 208.88,37.87 | 208.88,37.87 R39.2 | R9.CW 40,21.25 R4.2 41.74,27.79 C6.1 81.37,27.79 82.16,27 v82.16,15.12 | R46.1 179,77.04 v203.28,52.76 | v208.88,38.88 208.88,37.87
  Bottom 0.152: v203.28,52.76 208.88,47.16 v208.88,38.88 208.88,20.88 207.7,19.7 207.7,7.1 207.08,6.48 186.56,6.48 181.16,11.88 83.24,11.88 82.16,12.96 v82.16,15.12
N$7
  Top 0.152: SW1.12 221.25,18.14 R31.2
N$8
  Top 0.152: SW1.11 223.79,20.68 R30.2
N$9
  Top 0.152: SW1.10 226.33,20.68 R29.2
N$10
  Top 0.152: SW1.9 228.87,20.68 R28.2
N$11
  Top 0.152: SW1.8 231.41,20.68 R27.2
N$12
  Top 0.152: SW1.7 233.95,20.68 R26.2
N$13
  Top 0.152: SW1.6 203.47,18.14 R25.2
N$14
  Top 0.152: SW1.5 206.01,18.14 R24.2
N$15
  Top 0.152: SW1.4 208.55,18.14 R23.2
N$16
  Top 0.152: SW1.3 211.09,18.14 R22.2
N$17
  Top 0.152: SW1.2 213.63,18.14 R21.2
N$18  (via drill 0.25)
  Top 0.152: U1.5 207.64,33.87 C8.2 C9.2 211.99,33.84 v213.2,33.84 | v215,26.12 216.02,25.1 R20.2 216.17,18.14 SW1.D SW1.1
  Bottom 0.152: v215,26.12 215,32.04 v213.2,33.84
N$19  (via drill 0.25)
  Top 0.152: v179,148 R46.2
  Bottom 0.152: J2.UPR-CTR v179,148
N$20
  Top 0.152: R36.2 R39.1 206.81,35.97 U1.6
N$21
  Top 0.152: R15.1 37,54.05 R9.WIPER
N$22  (via drill 0.25)
  Top 0.152: v45.08,54.36 45,54.44 R17.1
  Bottom 0.152: R13.WIPER 69.31,24.48 53,24.48 45.08,32.4 v45.08,54.36
N$23
  Top 0.152: R13.CW 76.21,21.46 C6.2
N$24
  Bottom 0.152: SW5.UP1 164.08,13.68 158.12,13.68 155.59,16.21 SW4.UP1 151.55,17.19 149.12,14.76 141.92,14.76 135.8,20.88 134.12,20.88 SW2.COM
N$25  (via drill 0.25)
  Top 0.152: C7.2 R33.2 52.64,57.96 53.79,56.81 U3.1 55.4,57.45 R34.1 59.85,59.05 v60.2,59.4 | SW2.DOWN 129.35,24.81 125,29.16 107.36,29.16 v103.6,32.92
  Bottom 0.152: v103.6,32.92 73.88,62.64 61.28,62.64 60.2,61.56 v60.2,59.4
N$26  (via drill 0.25)
  Top 0.152: R37.1 64.75,55.8 64.52,55.8 64.26,55.54 U3.13 59.02,55.54 v58.76,55.8 | v58.04,60.84 57.11,60.84 R34.2
  Bottom 0.152: v58.76,55.8 58.76,60.12 v58.04,60.84
N$27  (1 unrouted)
  Top 0.152: R15.2 R16.1 | 45.01,57.96 45.8,57.96 47.71,56.05 C7.1 R33.1 51.51,55.54 U3.2
N$28  (via drill 0.25)
  Top 0.152: U3.14 62.65,56.81 63.26,57.42 | 63.26,57.42 63.8,57.96 R37.2 | "PID".TP 63,57.68 63.26,57.42 | SW2.UP 130.85,17.19 127.88,20.16 127.88,25.56 124.64,28.8 106.28,28.8 v102.16,32.92
  Bottom 0.152: v102.16,32.92 74.08,61 "PID".TP
N$29
  Top 0.152: U3.6 53.78,50.46 53,49.68 C5.1 52.95,47 52,47 50,45 50,39.24 | 50,39.24 56.6,39.24 57.85,37.99 U2.6 | R4.1 40,29.24 50,39.24
N$30  (via drill 0.25)
  Top 0.152: 55.52,46.8 53.77,45.05 C5.2 53,41 v53.72,40.28 | 55.52,46.8 55.85,46.8 R11.1 | U3.7 55.4,46.92 55.52,46.8 | U2.1 55.33,37.99 v54.8,38.52
  Bottom 0.152: v54.8,38.52 54.8,39.2 v53.72,40.28
N$31
  Top 0.152: R11.2 57.68,45.05 | 57.68,45.05 R19.1 | U3.9 58.46,50.46 57.68,49.68 57.68,45.05
N$32  (via drill 0.25)
  Top 0.152: R19.2 60.6,48.55 U3.8 63.08,49.19 | 63.08,49.19 64.76,49.19 R32.2 | "I".TP 63,49.11 63.08,49.19 | R14.CW 62.66,25.92 v62.72,25.92
  Bottom 0.152: v62.72,25.92 63.08,25.92 64.88,27.72 64.88,41.12 "I".TP
N$33  (via drill 0.25)
  Top 0.152: SW5.UP2 168.9,13.68 163.88,13.68 160.41,17.15 SW4.UP2 | R18.2 63.89,29.16 89.36,29.16 v92.6,25.92
  Bottom 0.152: SW5.UP2 167.46,12.24 97.64,12.24 96.56,13.32 96.56,21.96 v92.6,25.92
N$34  (via drill 0.25)
  Top 0.152: v41.84,54.36 42,54.52 R16.2
  Bottom 0.152: R14.WIPER 41.84,33.95 v41.84,54.36
N$35
  Top 0.152: 155.59,25.19 158.12,27.72 164.68,27.72 SW5.DN1 167.48,24.92 167.48,28.08 176,36.6 R47.1 | 155.59,25.19 SW4.DN1 | R41.WIPER 19,17.8 23.48,13.32 149.48,13.32 150.92,14.76 150.92,20.52 155.59,25.19
N$36  (via drill 0.25)
  Top 0.152: R42.CW 93.54,15.62 95.12,14.04 123.2,14.04 v123.56,14.4 | v152,14.4 152.72,15.12 152.72,20.16 153.56,21 SW4.COM1
  Bottom 0.152: v123.56,14.4 v152,14.4
N$37
  Top 0.152: U5.6 U5.7 139,49.37 139.76,48.6 139.76,34.71 R48.1
N$38  (via drill 0.25)
  Top 0.152: R42.WIPER 95.77,25.56 v112.04,25.56 | R44.1 118.88,33.93 v118.88,33.84
  Bottom 0.152: v118.88,33.84 112.04,27 v112.04,25.56
N$39
  Top 0.152: U5.5 137.32,52.05 C20.2 R44.2
N$40
  Top 0.152: 141.56,32.04 141.56,18.72 143.09,17.19 SW6.UP | 141.56,32.04 141.56,32.4 141.92,32.76 144.08,32.76 144.44,33.12 144.44,38.52 149.84,43.92 149.84,72.64 152.72,75.52 152.72,149.76 149,153.48 J3.UPR-CTR | R48.2 141.55,32.05 141.56,32.04
N$41
  Top 0.152: U2.3 55.83,33.12 R12.2 56.41,32.95 58.04,31.32 58.73,31.32 R10.1 59.57,31.05 61.28,32.76 61.81,32.76 R18.1
N$42
  Top 0.152: R40.2 111.32,53.95 | 111.32,53.95 R38.2 | U4.5 111.47,53.8 111.32,53.95
N$43  (via drill 0.25)
  Top 0.152: v162.44,14.4 156.68,14.4 v155.6,13.32
  Bottom 0.152: SW5.COM1 165.44,21 164.24,19.8 164.24,16.2 v162.44,14.4 | v155.6,13.32 154.88,12.6 114.2,12.6 111.54,15.26 R43.CW
N$44
  Top 0.152: U5.2 U5.1 143,47.63 R49.1
N$45  (via drill 0.25)
  Top 0.152: R43.WIPER 115.92,27.72 v121.76,27.72 | v146.96,42.84 147,42.88 R45.1
  Bottom 0.152: v121.76,27.72 134,39.96 144.8,39.96 146.96,42.12 v146.96,42.84
N$46
  Top 0.152: C22.2 147,50.76 | 147,50.76 R45.2 | U5.3 142.66,50.76 147,50.76
N$47
  Top 0.152: SW6.DOWN 146,29.05 145.16,29.89 145.16,32 | J3.LWR-CTR 149.13,156.96 152,156.96 153.44,155.52 153.44,75.52 150.2,72.28 150.2,43.2 145.16,38.16 145.16,32 | R49.2 145.11,32.05 145.16,32
N$48
  Top 0.152: R35.1 118.17,41.05 118.88,41.76 118.88,45.72 118.16,46.44 116.61,46.44 | 116.61,46.44 U4.2 | 116.61,46.44 114.92,46.44 114.56,46.8 114.56,50.61 C10.1
N$49
  Top 0.152: R41.CW 21.54,15.98 23.84,13.68 123.92,13.68 125,14.76 125,19.44 123.56,20.88 122.12,20.88 SW3.COM
N$50  (via drill 0.25)
  Top 0.152: v206,148 R6.1
  Bottom 0.152: J1.LWR-CTR 206.09,157.09 205,156 205,149 v206,148
N$51  (via drill 0.25)
  Top 0.152: C10.2 115.23,53.95 114.56,53.28 114.56,52.56 113.84,51.84 | 113.84,51.84 113.21,51.84 R38.1 | 113.84,51.84 113.84,46.44 115.19,45.09 U4.1 117.7,45.09 118.16,44.64 118.16,42.48 117.8,42.12 116,42.12 115.64,41.76 115.64,34.56 v118.52,31.68
  Bottom 0.152: v118.52,31.68 118.52,18.36 119.69,17.19 SW3.UP
N$52
  Top 0.152: R50.1 148.76,30.29 148.76,22.32 147.44,21 SW6.COM
N$53  (via drill 0.25)
  Top 0.152: R6.2 206,51.48 202.04,47.52 189.52,47.52 v171,29
  Bottom 0.152: v171,29 126.19,29 SW3.DOWN
N$54  (via drill 0.25)
  Top 0.152: v176,148 R47.2
  Bottom 0.152: J2.LWR-CTR 176.09,157.09 175,156 175,149 v176,148
N$55
  Top 0.152: R35.2 116.75,43.2 115.28,43.2 113.12,45.36 113.12,46.08 112.83,46.37 U4.7 109.95,46.37 109.52,46.8 109.52,51.57 R40.1 107.51,52.05 106.28,53.28 106.28,56.16 SCAN.TP
N$56
  Top 0.152: R50.2 M+.TP
N$57
  Top 0.152: D1.T'OTHER 76.87,46.55 76.4,46.08 65.97,46.08 R32.1
N$58
  Top 0.635: C17.1 66,79 | 66,79 12V-.P$1 | L2.1 68,77 66,79
N$59
  Top 0.635: U7.OUT+ 116.78,85.7 C28.+ 124.25,85.95 C29.2 133,85.95 L4.1
N$60
  Top 0.635: L3.2 89.05,79.65 C21.+ 90.25,78.95 C23.2 95,79.16 U7.IN+
N$61  (via drill 0.25)
  Top 0.25: 238.99,60.28 239.74,60.28 240.74,61.28 241.97,61.28 v241.98,61.27 | 238.99,60.28 238.28,60.28 v238.27,60.27 238.26,60.28 237.49,60.28 235.74,58.53 236.36,57.91 236.37,57.91 v236.51,57.77 236.61,57.66 v237.74,56.53 | 238.99,60.28 238.99,56.08 v239.99,56.08
N$62
  Top 0.635: C17.2 66,83 | 66,83 12V+.P$1 | L1.1 68,85 66,83
N$63
  Top 0.152: R52.2 R51.1 55.95,143.41 U6.4
N$64
  Top 0.635: U7.OUT- 111,82 112.7,80.3 C28.- 126,80.3 | C29.1 126.25,80.3 126,80.3 | L5.1 129.3,77 126,80.3
N$65
  Top 0.152: SW7.UP 33.7,133.75 R56.2
N$66
  Top 0.152: SW7.COM 29.84,136.92 42.68,136.92 46.36,133.24 53.92,133.24 56,131.16 J5.CONDUCTOR
N$67
  Top 0.152: J4.CONDUCTOR 45,149.95 R53.1 35.78,147.95 SW7.DOWN
N$68
  Top 0.152: R53.2 55.87,146.05 57.27,144.65 U6.5
N$69  (2 unrouted)
N$70
  Top 0.152: R55.2 C26.2 | R54.1 C26.2 | U6.11 58.54,151.7 58.88,152.04 58.88,152.83 C26.2
N$71
  Top 0.152: 24V-.P$1 C27.- 69.87,147.15 C32.1 | R55.1 60.95,153.57 61.04,153.48 61.04,153.09 C26.1 62.96,153 63.92,152.04 63.92,147.23 C32.1 | U6.6 58.54,145.22 59.6,146.28 62.97,146.28 C32.1
N$72  (via drill 0.25)
  Top 0.152: 24V+.P$1 C27.+ 66.37,145.25 C32.2 62.53,145.25 v62.48,145.2 | U6.14 54.73,150.6 | 54.73,150.6 54.73,152.68 R54.2 | v55.28,150.6 54.73,150.6
  Bottom 0.152: v62.48,145.2 60.68,145.2 v55.28,150.6
N$74
  Top 0.152: U6.3 54.73,141.41 54.2,140.88 54.2,140.15 R51.2 38.05,140 R56.1
N$223  (via drill 0.25)
  Top 0.25: v240.24,74.48 240.24,72.03 241.74,70.53 242.39,70.53 v242.44,70.58 | 242.99,75.53 242.99,73.83 v242.94,73.78 v242.94,72.98 242.94,72.83 242.99,72.78 242.99,72.03 243.99,72.03 244.04,72.08 v244.24,72.08 | 242.99,75.53 243.49,75.53 243.54,75.48 v243.64,75.48 | v241.74,73.08 241.74,75.28 241.99,75.53 242.99,75.53 | v242.44,70.58 242.49,70.63 242.49,72.33 v241.74,73.08 | v242.44,70.58 242.49,70.53 242.99,70.53 243.49,71.03 243.49,71.28 243.54,71.33 v243.54,71.38 | 241.86,72.96 v241.74,73.08
N$224  (via drill 0.25)
  Top 0.25: 244.24,56.53 241.49,56.53 241.47,56.52 v241.25,56.52
N$249  (via drill 0.25)
  Top 0.25: v239.74,59.54 239.74,57.53 240.36,56.91 240.36,56.89 v240.49,56.76
N$252  (via drill 0.25)
  Top 0.25: 244.36,60.53 243.49,60.53 243.48,60.54 v243.24,60.54
N$253  (via drill 0.25)
  Top 0.25: 244.24,61.78 244.24,61.28 243.24,61.28 243.24,61.53 243.23,61.54 v243.3,61.77
N$254
  Top 0.25: 237.74,61.78 239.24,61.78 239.24,62.03
N$256  (via drill 0.25)
  Top 0.25: v237.24,66.28 237.03,66.28 237.02,66.29 237.01,66.29 235.75,66.29 235.73,66.27 235.73,65.29 236.11,64.92 236.11,64.9 236.22,64.79 v236.23,64.79
N$257  (via drill 0.25)
  Top 0.25: v240.49,58.02 v240.49,58.03 240.49,60.28 242.24,60.28 242.74,60.78 242.74,61.53 242.51,61.76 v242.51,61.78
N$258  (via drill 0.25)
  Top 0.25: 241.99,62.03 239.74,62.03 239.74,61.03 237.24,61.03 235.36,59.16 235.36,59.15 v235.23,59.02
N$259  (via drill 0.25)
  Top 0.25: v237.73,59.53 237.61,59.41 236.74,58.53 238.49,56.78 238.49,55.52 243.99,55.52 v243.99,55.77
N$260  (via drill 0.25)
  Top 0.25: 244.11,55.03 238.11,55.03 235.23,57.91 v235.23,58
N$261  (via drill 0.25)
  Top 0.25: v244.24,64.52 244.24,64.78 v244.24,66.52 v244.24,66.53 244.24,67.9 243.99,68.16 243.86,68.16 v243.74,68.28 243.24,68.28 242.99,68 242.99,67.56
N$262  (via drill 0.25)
  Top 0.25: v243.74,72.98 v243.74,74.58
N$264  (via drill 0.25)
  Top 0.25: v235.74,64.25 235.48,64.28 v234.98,64.78 v234.99,64.79 234.99,66.28 235.84,67.13 243.49,67.13 243.49,65.88 | v243.23,64.28 243.49,64.54 243.49,65.88 | v238.49,66.01 238.64,65.88 243.49,65.88
N$267  (via drill 0.25)
  Top 0.25: 237.9,65.41 237.9,66.57 242.65,66.57 v242.69,66.54 | v236.49,65.53 236.61,65.41 237.9,65.41 | 237.9,65.41 242.35,65.41 v242.73,65.03
N$268  (via drill 0.25)
  Top 0.25: 238.74,75.53 v238.74,75.48 239.34,76.08 241.04,76.08 | v241.74,71.48 241.74,71.53 240.99,72.28 240.99,74.43 v241.04,74.48 240.99,74.53 240.99,76.03 241.04,76.08 | v243.24,76.28 243.14,76.28 242.94,76.08 241.04,76.08
N$270  (via drill 0.25)
  Top 0.25: v237.74,74.78 238.49,74.03 238.49,72.78 238.54,72.73 v238.54,72.68
N$271  (via drill 0.25)
  Top 0.25: v237.74,73.68 237.74,72.03 237.99,71.78 v238.44,71.78 238.99,71.78 239.24,72.03 239.24,74.78 v239.94,75.48
N$273  (via drill 0.25)
  Top 0.25: v242.64,76.68 v239.84,76.68
N$275  (via drill 0.25)
  Top 0.25: v244.54,73.08 244.54,73.23 244.49,73.28 244.49,75.43 v244.54,75.48 244.49,75.53 244.49,76.78 243.99,77.28 239.49,77.28 237.86,75.66 237.81,75.66 v237.74,75.58
N$276  (via drill 0.25)
  Top 0.25: v241.14,80.28 243.49,80.28 243.99,80.78 244.49,80.78
N$277  (via drill 0.25)
  Top 0.25: v237.74,80.58 v237.74,83.28
N$279  (via drill 0.25)
  Top 0.25: v237.84,84.58 237.84,84.63 239.74,86.53 244.24,86.53 244.54,86.23 v244.54,85.88
N$280  (via drill 0.25)
  Top 0.25: v238.74,82.38 238.74,84.53 239.99,85.78 v243.64,85.78
N$281  (via drill 0.25)
  Top 0.25: v243.84,84.98 243.79,84.98 243.74,85.03 240.24,85.03 239.34,84.13 v239.34,81.88
N$283  (via drill 0.25)
  Top 0.152: v239.74,81.18 238.74,81.18 238.49,80.93 238.49,79.83
  Top 0.25: v238.04,79.78 238.54,79.78 | 238.54,79.78 v239.24,79.78 | 238.49,79.83 238.54,79.78
N$284  (via drill 0.25)
  Top 0.25: 240.24,80.38 240.24,80.53 240.74,81.03 243.24,81.03 243.29,81.08 v243.34,81.08 | 240.24,80.38 240.24,80.03 240.74,79.53 243.74,79.53 244.29,80.08 v244.34,80.08 | v239.05,80.48 239.09,80.43 240.19,80.43 240.24,80.38
WS-COM
  pour Top: 11.36,169.68 11.36,116.04 84.8,116.04 84.8,169.68
  pour Bottom: 11.36,169.68 11.36,116.04 84.8,116.04 84.8,169.68

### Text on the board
Top: Design By
tNames: WS3054 Amp / UofT - Physics | Loch Box Rev: A / University of Toronto / A. Steinberg Labs
Document: N.B.: In the library, temporarily remove the 4 lower mtg posts on the case.
Target: Alan
Graphics: 60.07 / ref | 0.506" / 6 pl | 1/4" | 29.06 | 3/16" | 13.06 | 0 | 0 | 100 | 150.5 | 180.5 | 210.5 | 254 / ref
